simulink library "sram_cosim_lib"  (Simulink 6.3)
undefined symbols (not defined in the file or in its folder): no_bitstream
libraries: xbsIndex_r4 x9, sram_cosim_lib x1

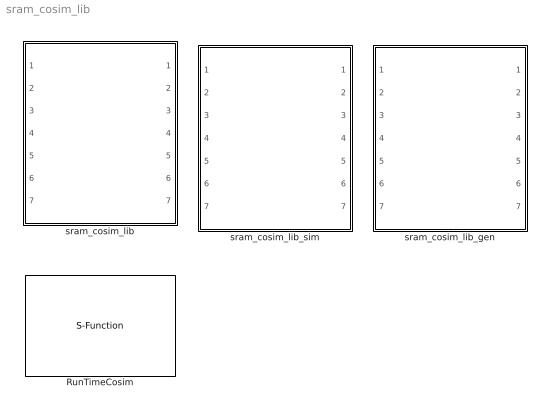
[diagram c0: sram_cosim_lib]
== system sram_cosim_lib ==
  RunTimeCosim : S-Function  FunctionName=adcosim  Parameters='d,in,unsigned,16,0;a,in,unsigned,8,0;w,in,boolean,1,0;r,in,boolean,1,0;q,out,unsigned,16,0;qv,out,boolean,1,0;',index,bitstream,freq,single_step,shared  mask{index=0, bitstream=no_bitstream, freq=50, single_step=off, shared=None}
      mask prompts: index "Card Index"; freq "Clock Frequency"; single_step "Single Step"; shared "Share Access"
  sram_cosim_lib : Subsystem  Tag=configX  BlockChoice=sram_cosim_lib_sim
  sram_cosim_lib_gen : Subsystem
  sram_cosim_lib_sim : Subsystem

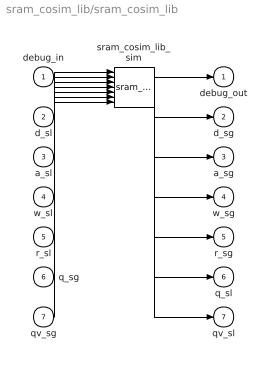
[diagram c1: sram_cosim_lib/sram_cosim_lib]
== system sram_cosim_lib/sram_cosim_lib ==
  debug_in : Inport
  d_sl : Inport  Port=2
  a_sl : Inport  Port=3
  w_sl : Inport  Port=4
  r_sl : Inport  Port=5
  q_sg : Inport  Port=6
  qv_sg : Inport  Port=7
  sram_cosim_lib_sim : sram_cosim_lib/sram_cosim_lib_sim
  debug_out : Outport
  d_sg : Outport  Port=2
  a_sg : Outport  Port=3
  w_sg : Outport  Port=4
  r_sg : Outport  Port=5
  q_sl : Outport  Port=6
  qv_sl : Outport  Port=7
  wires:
  debug_in/1 -> sram_cosim_lib_sim/1
  d_sl/1 -> sram_cosim_lib_sim/2
  a_sl/1 -> sram_cosim_lib_sim/3
  w_sl/1 -> sram_cosim_lib_sim/4
  r_sl/1 -> sram_cosim_lib_sim/5
  q_sg/1 -> sram_cosim_lib_sim/6
  qv_sg/1 -> sram_cosim_lib_sim/7
  sram_cosim_lib_sim/1 -> debug_out/1
  sram_cosim_lib_sim/2 -> d_sg/1
  sram_cosim_lib_sim/3 -> a_sg/1
  sram_cosim_lib_sim/4 -> w_sg/1
  sram_cosim_lib_sim/5 -> r_sg/1
  sram_cosim_lib_sim/6 -> q_sl/1
  sram_cosim_lib_sim/7 -> qv_sl/1

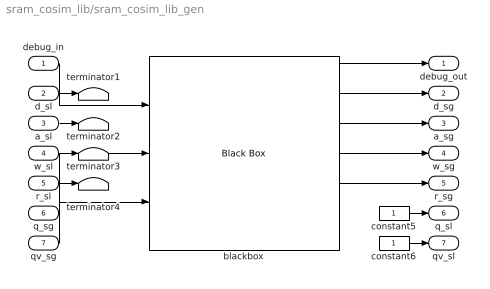
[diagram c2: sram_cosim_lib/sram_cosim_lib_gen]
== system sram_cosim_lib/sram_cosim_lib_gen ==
  debug_in : Inport
  d_sl : Inport  Port=2
  a_sl : Inport  Port=3
  w_sl : Inport  Port=4
  r_sl : Inport  Port=5
  q_sg : Inport  Port=6
  qv_sg : Inport  Port=7
  blackbox : xbsIndex_r4/Black Box  init_code=sram_cosim_lib_config  sim_method=Inactive  block_type=blackbox2
  constant5 : Constant
  constant6 : Constant
  terminator{1..4} (4 alike) : Terminator
  debug_out : Outport
  d_sg : Outport  Port=2
  a_sg : Outport  Port=3
  w_sg : Outport  Port=4
  r_sg : Outport  Port=5
  q_sl : Outport  Port=6
  qv_sl : Outport  Port=7
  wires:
  d_sl/1 -> terminator1/1
  a_sl/1 -> terminator2/1
  w_sl/1 -> terminator3/1
  r_sl/1 -> terminator4/1
  constant5/1 -> q_sl/1
  constant6/1 -> qv_sl/1
  debug_in/1 -> blackbox/1
  blackbox/1 -> debug_out/1
  blackbox/2 -> d_sg/1
  blackbox/3 -> a_sg/1
  blackbox/4 -> w_sg/1
  blackbox/5 -> r_sg/1
  q_sg/1 -> blackbox/2
  qv_sg/1 -> blackbox/3

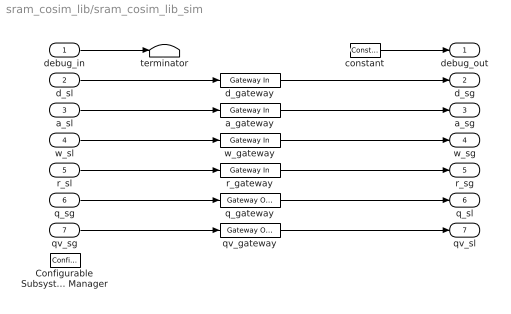
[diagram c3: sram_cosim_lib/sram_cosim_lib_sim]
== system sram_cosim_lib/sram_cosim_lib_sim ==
  debug_in : Inport
  d_sl : Inport  Port=2
  a_sl : Inport  Port=3
  w_sl : Inport  Port=4
  r_sl : Inport  Port=5
  q_sg : Inport  Port=6
  qv_sg : Inport  Port=7
  Configurable Subsystem Manager : xbsIndex_r4/Configurable Subsystem Manager  Tag=xcfgMgr  block_type=configsubsys
  a_gateway : xbsIndex_r4/Gateway In  arith_type=Unsigned  n_bits=8  bin_pt=0  period=1  dbl_ovrd=off  timing_constraint=None  locs_specified=off  LOCs={}  block_type=gatewayin
  constant : xbsIndex_r4/Constant  arith_type=Unsigned  const=1  n_bits=32  bin_pt=0  explicit_period=on  period=1  equ=P=C  opselect=C  inp2=PCIN>>17  opr=+  inp1=P  carry=CIN  dbl_ovrd=off  block_type=constant
  d_gateway : xbsIndex_r4/Gateway In  arith_type=Unsigned  n_bits=16  bin_pt=0  period=1  dbl_ovrd=off  timing_constraint=None  locs_specified=off  LOCs={}  block_type=gatewayin
  q_gateway : xbsIndex_r4/Gateway Out  hdl_port=on  timing_constraint=None  locs_specified=off  LOCs={}  block_type=gatewayout
  qv_gateway : xbsIndex_r4/Gateway Out  hdl_port=on  timing_constraint=None  locs_specified=off  LOCs={}  block_type=gatewayout
  r_gateway : xbsIndex_r4/Gateway In  arith_type=Boolean  n_bits=1  bin_pt=0  period=1  dbl_ovrd=off  timing_constraint=None  locs_specified=off  LOCs={}  block_type=gatewayin
  terminator : Terminator
  w_gateway : xbsIndex_r4/Gateway In  arith_type=Boolean  n_bits=1  bin_pt=0  period=1  dbl_ovrd=off  timing_constraint=None  locs_specified=off  LOCs={}  block_type=gatewayin
  debug_out : Outport
  d_sg : Outport  Port=2
  a_sg : Outport  Port=3
  w_sg : Outport  Port=4
  r_sg : Outport  Port=5
  q_sl : Outport  Port=6
  qv_sl : Outport  Port=7
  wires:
  debug_in/1 -> terminator/1
  constant/1 -> debug_out/1
  d_sl/1 -> d_gateway/1
  d_gateway/1 -> d_sg/1
  a_sl/1 -> a_gateway/1
  a_gateway/1 -> a_sg/1
  w_sl/1 -> w_gateway/1
  w_gateway/1 -> w_sg/1
  r_sl/1 -> r_gateway/1
  r_gateway/1 -> r_sg/1
  q_sg/1 -> q_gateway/1
  q_gateway/1 -> q_sl/1
  qv_sg/1 -> qv_gateway/1
  qv_gateway/1 -> qv_sl/1
